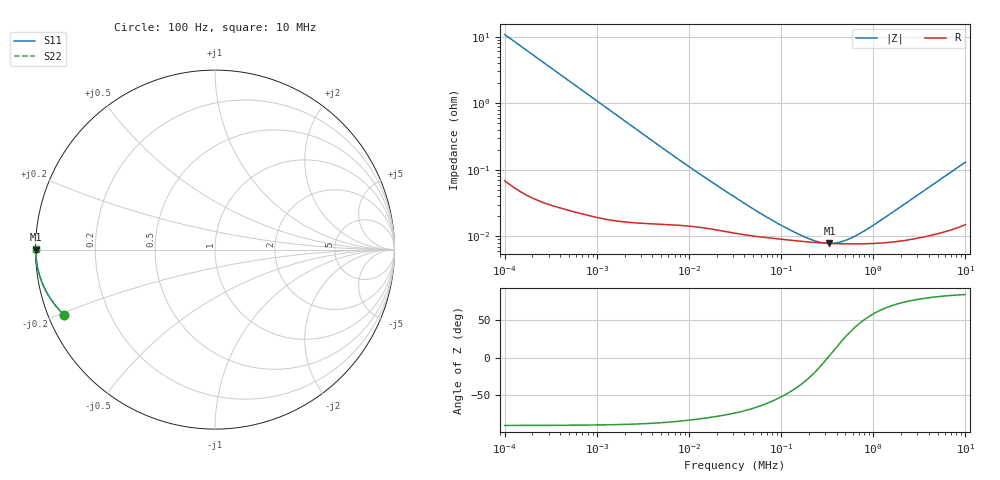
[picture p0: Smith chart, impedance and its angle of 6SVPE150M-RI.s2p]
!  *** S-Parameter ***
!  Copyright (C) Panasonic Industry
!  Conductive Polymer Aluminum Solid Capacitors (OS-CON)
!  Parts No. 6SVPE150M
! Touchstone file from project
# GHZ S RI R 50.000000
! Modal data exported
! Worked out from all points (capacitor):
!   401 points, 100 Hz to 10 MHz, reference 50 ohm
!   read as one part in shunt: C = 147 uF near 105.9 Hz
!   lowest |Z| = 7.86 mohm at 335 kHz (marker M1)
!   series resonance near 321.8 kHz, so ESL is about 1.7 nH
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1e-07  -0.8415 -0.3621  0.1585 -0.3621  0.1585 -0.3621  -0.8415 -0.3621
! Port Impedance 5.000000E+001 0.000000E+000 5.000000E+001 0.000000E+000
1.059254e-07  -0.8561 -0.3479  0.1439 -0.3479  0.1439 -0.3479  -0.8561 -0.3479
1.453784e-07  -0.9174 -0.272  0.0826 -0.272  0.0826 -0.272  -0.9174 -0.272
2.113489e-07  -0.9586 -0.1957  0.0414 -0.1957  0.0414 -0.1957  -0.9586 -0.1957
3.651741e-07  -0.9851 -0.1166  0.0149 -0.1166  0.0149 -0.1166  -0.9851 -0.1166
6.878599e-07  -0.9952 -0.0627  0.00482 -0.0627  0.00482 -0.0627  -0.9952 -0.0627
1.539927e-06  -0.9985 -0.0282  0.00149 -0.0282  0.00149 -0.0282  -0.9985 -0.0282
4.731513e-06  -0.9993 -0.00923  0.000696 -0.00923  0.000696 -0.00923  -0.9993 -0.00923
1.188502e-05  -0.9994 -0.00376  0.000571 -0.00376  0.000571 -0.00376  -0.9994 -0.00376
3.162278e-05  -0.9996 -0.00148  0.000449 -0.00148  0.000449 -0.00148  -0.9996 -0.00148
5.78762e-05  -0.9996 -0.000821  0.000396 -0.000821  0.000396 -0.000821  -0.9996 -0.000821
9.440609e-05  -0.9996 -0.000493  0.000366 -0.000493  0.000366 -0.000493  -0.9996 -0.000493
0.0001539927  -0.9997 -0.000267  0.000341 -0.000267  0.000341 -0.000267  -0.9997 -0.000267
0.0002175204  -0.9997 -0.000137  0.000326 -0.000137  0.000326 -0.000137  -0.9997 -0.000137
0.000273842  -0.9997 -5.61e-05  0.000319 -5.61e-05  0.000319 -5.61e-05  -0.9997 -5.61e-05
0.0003349654  -0.9997 1.41e-05  0.000314 1.41e-05  0.000314 1.41e-05  -0.9997 1.41e-05
0.0004466836  -0.9997 0.000118  0.00031 0.000118  0.00031 0.000118  -0.9997 0.000118
0.0005956621  -0.9997 0.000233  0.000309 0.000233  0.000309 0.000233  -0.9997 0.000233
0.0008659643  -0.9997 0.000414  0.000311 0.000414  0.000311 0.000414  -0.9997 0.000414
0.001496236  -0.9997 0.000789  0.000326 0.000789  0.000326 0.000789  -0.9997 0.000789
0.009440609  -0.9994 0.00491  0.000605 0.00491  0.000605 0.00491  -0.9994 0.00491
0.01  -0.9994 0.00519  0.000628 0.00519  0.000628 0.00519  -0.9994 0.00519
